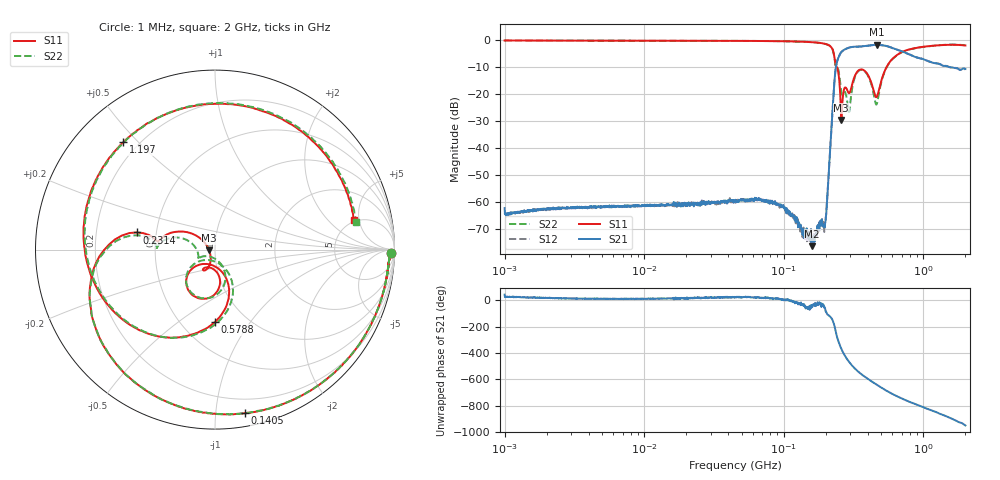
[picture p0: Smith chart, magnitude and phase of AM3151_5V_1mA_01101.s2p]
! Date/Time: Fri Jun 26 10:41:14 2020
! Network Analyzer:  Rev:
! Sweep from 1000000.0 to 2000000000.0, 1601 Points ! Power Supply: 0 V, 0 A
# HZ S DB R 50
!freq MagS11 AngS11 MagS21 AngS21 MagS12 AngS12 MagS22 AngS22
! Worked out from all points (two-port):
!   1601 points, 1 MHz to 2 GHz, reference 50 ohm
!   highest |S21| = -1.76 dB at 463 MHz (marker M1); lowest = -76.3 dB at 159.7 MHz (marker M2)
!   |S21| within 3 dB of the highest: 255.8 MHz to 747.6 MHz (491.8 MHz wide, 98 % of centre)
!   lowest |S11| = -29.6 dB at 258.1 MHz (marker M3), VSWR 1.07, Z = 46.8 - j0.319 ohm
!   |S11| at or under -10 dB: 239.6 MHz to 545 MHz (305.4 MHz wide, 77.9 % of centre)
!   |S22| runs from -26.7 to -0.2 dB; largest |S21 - S12| = 0.0076
!   S11 on the Smith chart (normalised r, x): 1 MHz: 56, -52; 140.5 MHz: 0.09, -1.20; 231.4 MHz: 0.39, +0.09; 578.8 MHz: 0.72, -0.69; 1.197 GHz: 0.14, +0.45; 2 GHz: 4.82, +4.22
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1000000  -0.17 -1.0  -62.21 45.3  -64.11 25.8  -0.17 -1.0
3555161  -0.23 -2.3  -61.74 15.1  -61.69 13.3  -0.23 -2.3
1.263916e7  -0.27 -6.9  -61.05 14.8  -61.22 14.5  -0.27 -6.9
4.493426e7  -0.32 -24.0  -59.40 24.7  -59.80 24.2  -0.32 -24.0
9.746975e7  -0.44 -53.1  -61.62 5.7  -61.10 8.0  -0.45 -52.9
1.405178e8  -0.66 -79.6  -70.51 -34.0  -70.23 -43.1  -0.65 -79.4
1.589914e8  -0.79 -92.5  -75.25 -46.6  -72.35 -38.3  -0.81 -92.4
1.597485e8  -0.82 -93.1  -76.27 -51.3  -74.87 -52.3  -0.82 -92.9
1.978234e8  -1.42 -128.0  -67.66 -63.7  -66.53 -63.0  -1.43 -127.9
2.313992e8  -7.01 167.6  -14.31 159.9  -14.30 159.9  -7.24 169.4
2.449739e8  -11.53 159.5  -6.79 55.9  -6.82 55.9  -10.64 170.5
2.581155e8  -29.59 -174.1  -4.49 -7.1  -4.49 -7.2  -19.22 174.0
2.879163e8  -19.08 -116.8  -2.97 -95.5  -2.95 -95.5  -24.62 -141.4
3.351872e8  -11.77 -92.5  -2.45 -174.3  -2.45 -174.4  -12.02 -87.7
3.995981e8  -12.80 -134.2  -2.11 123.6  -2.12 123.4  -13.08 -136.3
4.63e8  -21.08 -100.1  -1.76 78.3  -1.78 78.2  -23.75 -95.6
5.652395e8  -8.63 -85.1  -2.47 22.3  -2.48 22.2  -8.75 -81.6
5.788261e8  -7.90 -90.0  -2.66 16.4  -2.64 16.3  -7.99 -86.8
8.75068e8  -2.97 -170.7  -6.28 -69.4  -6.26 -69.4  -3.03 -171.9
1.197317e9  -2.09 130.5  -8.54 -124.7  -8.49 -124.5  -2.08 127.7
1.554828e9  -1.75 75.3  -10.05 -174.6  -10.09 -175.4  -1.70 72.4
2e9  -2.03 11.9  -10.72 128.1  -10.89 127.6  -1.92 10.9
